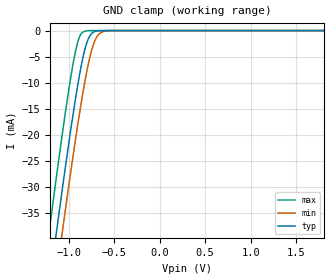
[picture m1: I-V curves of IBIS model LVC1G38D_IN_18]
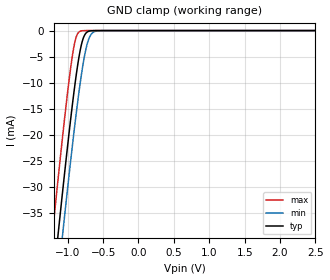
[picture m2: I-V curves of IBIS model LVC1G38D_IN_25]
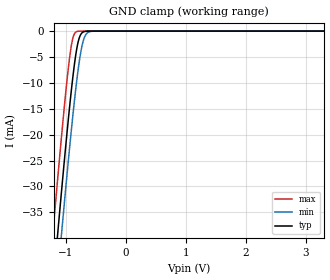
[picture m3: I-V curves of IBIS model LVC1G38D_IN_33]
| TEXAS INSTRUMENTS INCORPORATED
| Standard Linear and Logic Group
| IBIS Model of SN74LVC1G38
| Single 2-Input Nand Gate with Open Drain Output
| This file contains package information for the following:
|  SOT 5-pin (DCK) package as [Component] LVC1G38D_DCK
|  SOT 5-pin (DBV) package as [Component] LVC1G38D_DBV
|  DSBGA 5-pin (YEP) package as [Component] LVC1G38D_YEP
|  DSBGA 5-pin (YZP) package as [Component] LVC1G38D_YZP
|  SON 5-pin (DPW) package as [Component] LVC1G38D_DPW
| This device can be powered at the following Vccs:
|  1.8 volt Vcc
|  2.5 volt Vcc
|  3.3 volt Vcc
|  5 volt Vcc
| This file provides unique models under the [Model Selector] for each Vcc.
| For operation at a specific Vcc, select the appropriate model after each
| [Model Selector] keyword.
[IBIS Ver]   4.1
[Comment char]  |_char
[File Name]   sn74lvc1g38.ibs
[File Rev]   1.3 | x_die
[Date]   August 17, 2017
[Source]   Data created from TI-SPICE simulations at TI-SLL.
[Notes]   The following is an IBIS list for the LVC1G38.
   Please contact sllibis@ti.com with questions and
   comments concerning SLL IBIS models.
   - FILE REV HISTORY
   - 1.1 Release IBIS file on 10/02/03
   - 1.2 YEP and YZP packages released on 06/29/04
   - 1.3 DPW package component added
   - Power-clamp data has been deleted since there is no
   power-clamp diode in the device.
[Disclaimer]  This model is designed as an aid for customers of Texas Instruments
 TI and its licensors and suppliers make no warranties, either expressed
 or implied, with respect to this  model, including the warranties of
 merchantability or fitness for a particular purpose.
 The model is provided solely on an "as is" basis. The entire risk as to
 its quality and performance is with the customer.
[Copyright] (C)Copyright 2017 Texas Instruments Incorporated.
   All rights reserved.
| Component LVC1G38D_DCK 5-pin SOT
[Component]   LVC1G38D_DCK
[Manufacturer]   Texas Instruments, Inc.
[Package]
|   typ   min   max
R_pkg   2.000e-02   1.700e-02   2.500e-02
L_pkg   9.980e-10   8.810e-10   1.069e-09
C_pkg   1.460e-13   1.180e-13   2.050e-13
[Pin]   signal_name   model_name   R_pin   L_pin   C_pin
1   A   LVC1G38D_IN   1.900e-02   1.069e-09   1.620e-13
2   B   LVC1G38D_IN   1.800e-02   8.810e-10   1.210e-13
3   GND   GND   1.700e-02   1.031e-09   2.050e-13
4   Y   LVC1G38D_OUT   2.000e-02   9.600e-10   1.240e-13
5   VCC   POWER   2.500e-02   1.049e-09   1.180e-13
| Component LVC1G38D_DBV 5-pin SOT
[Component]   LVC1G38D_DBV
[Manufacturer]   Texas Instruments, Inc.
[Package]
|   typ   min   max
R_pkg   2.500e-02   2.100e-02   2.900e-02
L_pkg   1.529e-09   1.312e-09   1.906e-09
C_pkg   1.560e-13   1.100e-13   2.400e-13
[Pin]   signal_name   model_name   R_pin   L_pin   C_pin
1   A   LVC1G38D_IN   2.100e-02   1.511e-09   1.440e-13
2   B   LVC1G38D_IN   2.300e-02   1.312e-09   1.380e-13
3   GND   GND   2.900e-02   1.906e-09   2.400e-13
4   Y   LVC1G38D_OUT   2.600e-02   1.541e-09   1.500e-13
5   VCC   POWER   2.500e-02   1.374e-09   1.100e-13
| Component LVC1G38D_YEP 5-pin DSBGA
[Component]   LVC1G38D_YEP
[Manufacturer]   Texas Instruments, Inc.
[Package]
|   typ   min   max
R_pkg   1.000e-03   1.000e-03   1.000e-03
L_pkg   2.500e-11   2.500e-11   2.500e-11
C_pkg   6.340e-14   6.200e-14   6.500e-14
[Pin]   signal_name   model_name   R_pin   L_pin   C_pin
1   A   LVC1G38D_IN   1.000e-03   2.500e-11   6.400e-14
2   B   LVC1G38D_IN   1.000e-03   2.500e-11   6.500e-14
3   GND   GND   1.000e-03   2.500e-11   6.400e-14
4   Y   LVC1G38D_OUT   1.000e-03   2.500e-11   6.200e-14
5   VCC   POWER   1.000e-03   2.500e-11   6.200e-14
| Component LVC1G38D_YZP 5-pin DSBGA
[Component]   LVC1G38D_YZP
[Manufacturer]   Texas Instruments, Inc.
[Package]
|   typ   min   max
R_pkg   1.000e-03   1.000e-03   1.000e-03
L_pkg   2.500e-11   2.500e-11   2.500e-11
C_pkg   6.340e-14   6.200e-14   6.500e-14
[Pin]   signal_name   model_name   R_pin   L_pin   C_pin
1   A   LVC1G38D_IN   1.000e-03   2.500e-11   6.400e-14
2   B   LVC1G38D_IN   1.000e-03   2.500e-11   6.500e-14
3   GND   GND   1.000e-03   2.500e-11   6.400e-14
4   Y   LVC1G38D_OUT   1.000e-03   2.500e-11   6.200e-14
5   VCC   POWER   1.000e-03   2.500e-11   6.200e-14
| Component LVC1G38D_DPW 5-pin X2SON
[Component]   LVC1G38D_DPW
[Manufacturer]   Texas Instruments, Inc.
[Package]
|   typ   min   max
R_pkg   0.0364   0.0010   0.0518
L_pkg   0.2978n   0.0346n   0.4435n
C_pkg   0.0978p   0.0741p   0.1133p
[Pin]   signal_name   model_name   R_pin   L_pin   C_pin
1   D   LVC1G38D_IN   0.04116   0.30011n   0.10160p
2   CLK   LVC1G38D_IN   0.05181   0.44351n   0.11332p
3   GND   GND   0.00103   0.03456n   0.07412p
4   Q   LVC1G38D_OUT   0.04142   0.34311n   0.10148p
5   VCC   POWER   0.04662   0.36767n   0.09844p
| Model LVC1G38D_IN
[Model Selector]   LVC1G38D_IN
LVC1G38D_IN_18   1.8 volt Vcc
LVC1G38D_IN_25   2.5 volt Vcc
LVC1G38D_IN_33   3.3 volt Vcc
LVC1G38D_IN_50   5 volt Vcc
| Model LVC1G38D_OUT
[Model Selector]   LVC1G38D_OUT
LVC1G38D_OUT_18   1.8 volt Vcc
LVC1G38D_OUT_25   2.5 volt Vcc
LVC1G38D_OUT_33   3.3 volt Vcc
LVC1G38D_OUT_50   5 volt Vcc
| Models and submodels in the file (8): LVC1G38D_IN_18 (Input), LVC1G38D_IN_25 (Input), LVC1G38D_IN_33 (Input), LVC1G38D_IN_50 (Input), LVC1G38D_OUT_18 (Open_drain), LVC1G38D_OUT_25 (Open_drain), LVC1G38D_OUT_33 (Open_drain), LVC1G38D_OUT_50 (Open_drain)
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[Model]   LVC1G38D_IN_18
Model_type  Input
Vinl=0.5775
Vinh=1.2675
| variable   typ   min   max
C_comp   3.50pF   3.04pF   4.31pF
[Temperature Range]   40   100   -40
| Ambient temperature   25   85   -40
[Voltage range]   1.8   1.65   1.95
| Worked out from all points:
|   GND clamp passes 1 mA (typ) near -0.77 V on its own axis
[GND Clamp]
| LVC1G38D_IN_18
|   Voltage   I(typ)   I(min)   I(max)
-5.5V     -655.2mA   -662.2mA   -646.6mA
-1.215V   -49.6mA    -57.88mA   -38.96mA
-1.135V   -39.07mA   -47.36mA   -28.42mA
-1.075V   -31.35mA   -39.6mA    -20.75mA
-1.055V   -28.82mA   -37.05mA   -18.27mA
-955mV    -16.68mA   -24.66mA   -6.874mA
-885mV    -9.098mA   -16.55mA   -1.486mA
-825mV    -3.922mA   -10.26mA   -137.1uA
-780mV    -1.472mA   -6.227mA   -17.15uA
-715mV    -205.4uA   -2.128mA   -808.5nA
-650mV    -22.01uA   -443.9uA   -37.93nA
1.8V      3.326pA    6.142pA    3.026pA
[Model]   LVC1G38D_IN_25
Model_type  Input
Vinl=0.7
Vinh=1.7
| variable   typ   min   max
C_comp   3.43pF   2.83pF   4.39pF
[Temperature Range]   40   100   -40
| Ambient temperature   25   85   -40
[Voltage range]   2.5   2.3   2.7
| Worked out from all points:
|   GND clamp passes 1 mA (typ) near -0.77 V on its own axis
[GND Clamp]
| LVC1G38D_IN_25
|   Voltage   I(typ)   I(min)   I(max)
-5.5V     -655.2mA   -662.2mA   -646.6mA
-1.215V   -49.6mA    -57.88mA   -38.96mA
-1.14V    -39.72mA   -48.01mA   -29.07mA
-1.12V    -37.12mA   -45.41mA   -26.48mA
-1.08V    -31.98mA   -40.25mA   -21.38mA
-1.06V    -29.44mA   -37.69mA   -18.89mA
-960mV    -17.26mA   -25.26mA   -7.377mA
-890mV    -9.597mA   -17.1mA    -1.734mA
-785mV    -1.671mA   -6.635mA   -21.67uA
-720mV    -242.5uA   -2.354mA   -1.023uA
-650mV    -22.01uA   -443.9uA   -37.93nA
2.5V      4.713pA    7.577pA    4.389pA
[Model]   LVC1G38D_IN_33
Model_type  Input
Vinl=0.8
Vinh=2.0
| variable   typ   min   max
C_comp   3.35pF   2.67pF   4.41pF
[Temperature Range]   40   100   -40
| Ambient temperature   25   85   -40
[Voltage range]   3.3   3   3.6
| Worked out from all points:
|   GND clamp passes 1 mA (typ) near -0.77 V on its own axis
[GND Clamp]
| LVC1G38D_IN_33
|   Voltage   I(typ)   I(min)   I(max)
-5.5V     -655.2mA   -662.2mA   -646.6mA
-1.225V   -50.93mA   -59.21mA   -40.3mA
-1.145V   -40.37mA   -48.66mA   -29.72mA
-1.12V    -37.12mA   -45.41mA   -26.48mA
-1.08V    -31.98mA   -40.25mA   -21.38mA
-1.06V    -29.44mA   -37.69mA   -18.89mA
-965mV    -17.84mA   -25.87mA   -7.89mA
-885mV    -9.098mA   -16.55mA   -1.486mA
-780mV    -1.472mA   -6.227mA   -17.15uA
-715mV    -205.4uA   -2.128mA   -808.5nA
-640mV    -15.53uA   -338.1uA   -23.69nA
3.3V      6.304pA    9.258pA    5.93pA
